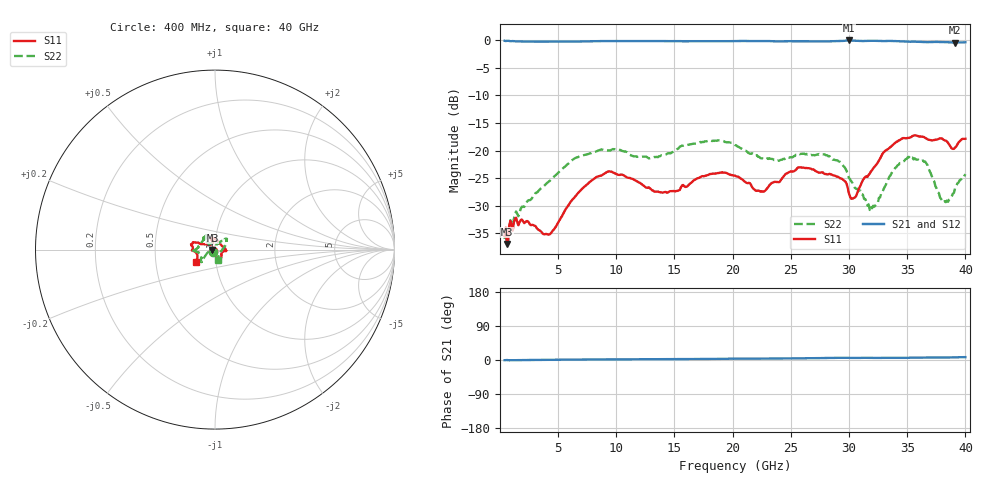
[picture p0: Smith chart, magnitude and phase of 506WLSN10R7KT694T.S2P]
!  American Technical Ceramics  Date:  8/31/2012
!  One Norden Lane
!  Huntington Station,  NY.  11746-2102
!  Tel:  (631) 622-4700  Fax:  (631) 622-4748
!  Part Number  506WLSN10R7KG694T
!  Description:  Ultra-Broadband Inductor
!  Application:  Ultra-broadband DC block decoupling, bias tee
# GHZ S DB R 50
! Freq  |S11|  S11 Ph  |S21|  S21 Ph  |S12|  S12 Ph  |S22|  S22 Ph
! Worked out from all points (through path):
!   401 points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, 400 MHz to 40 GHz, reference 50 ohm
!   highest |S21| = -0.03 dB at 30 GHz (marker M1); lowest = -0.4 dB at 39.11 GHz (marker M2)
!   lowest |S11| = -37.0 dB at 598 MHz (marker M3), VSWR 1.03, Z = 48.6 - j0.177 ohm
!   |S11| at or under -10 dB: start of sweep to end of sweep
!   |S22| runs from -37.4 to -18.1 dB; largest |S21 - S12| = 0.0079
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0.4  -35.47 -144.2  -0.09 -0.6  -0.11 -0.6  -36.05 -137.6
0.598  -36.95 -172.6  -0.10 -0.1  -0.12 -0.1  -37.36 -167.6
1.489  -33.01 -173.5  -0.20 -0.2  -0.21 -0.2  -31.49 -162.1
4.261  -35.22 -132.5  -0.24 0.5  -0.25 0.6  -25.54 -153.3
7.033  -27.00 -75.8  -0.22 1.3  -0.21 1.4  -20.95 -142.4
9.409  -23.79 -61.4  -0.13 1.5  -0.11 1.6  -20.01 -137.8
13.666  -27.53 -27.1  -0.14 1.8  -0.12 1.8  -21.06 -164.9
17.824  -24.47 -8.6  -0.18 2.7  -0.16 2.6  -18.29 -175.7
20.2  -24.55 1.8  -0.14 3.5  -0.12 3.3  -19.01 -179.1
22.576  -27.49 49.0  -0.14 3.7  -0.13 3.5  -21.47 155.7
25.645  -23.06 102.1  -0.18 4.4  -0.17 4.1  -20.58 122.4
26.833  -23.44 104.5  -0.19 4.6  -0.19 4.3  -20.85 126.6
29.11  -24.85 108.8  -0.15 5.8  -0.14 5.5  -21.98 140.9
30.001  -27.84 105.8  -0.03 5.6  -0.03 5.3  -25.00 136.2
30.496  -28.53 131.5  -0.08 5.3  -0.08 5.0  -26.76 139.0
31.981  -23.56 153.4  -0.09 5.6  -0.10 5.2  -30.48 83.6
33.466  -19.54 158.3  -0.13 5.7  -0.14 5.3  -24.75 53.4
35.248  -17.65 166.2  -0.27 6.1  -0.29 5.6  -20.94 42.1
36.535  -17.69 170.3  -0.33 6.2  -0.35 5.8  -21.99 34.1
38.119  -18.05 -178.0  -0.31 6.5  -0.34 6.2  -29.42 -18.8
39.109  -19.49 -157.4  -0.41 7.0  -0.43 6.7  -26.89 -64.6
40  -17.86 -148.0  -0.36 7.6  -0.37 7.2  -24.29 -74.7
